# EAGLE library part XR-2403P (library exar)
Enhanced MNP-5 modem MICROCONTROLLER
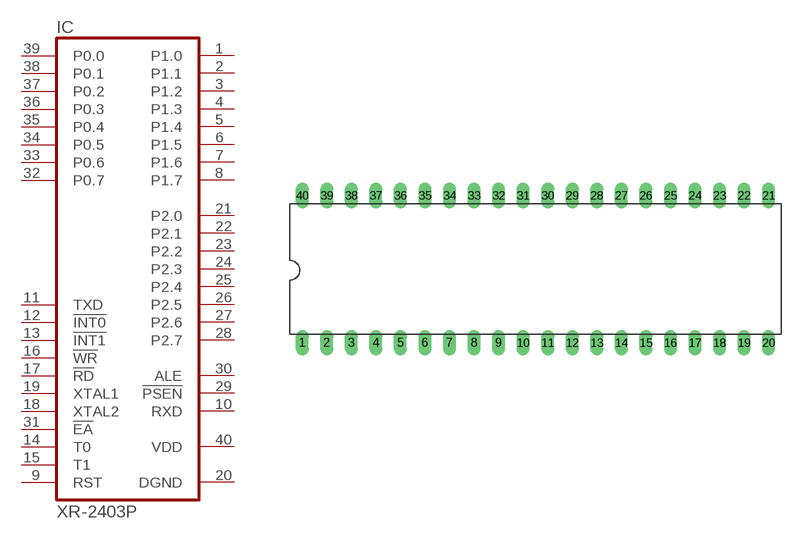
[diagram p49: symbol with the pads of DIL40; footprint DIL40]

Designator prefix IC

## XR-2403P (OC_FARNELL: unknown; OC_NEWARK: unknown)  [DIL40]
1  P1.0
2  P1.1
3  P1.2
4  P1.3
5  P1.4
6  P1.5
7  P1.6
8  P1.7
9  RST  in
10  RXD  out
11  TXD  in
12  !INT0  in
13  !INT1  in
14  T0  in
15  T1  in
16  !WR  in
17  !RD  in
18  XTAL2  in
19  XTAL1  in
20  DGND  pwr
21  P2.0
22  P2.1
23  P2.2
24  P2.3
25  P2.4
26  P2.5
27  P2.6
28  P2.7
29  !PSEN  out
30  ALE  out
31  !EA  in
32  P0.7
33  P0.6
34  P0.5
35  P0.4
36  P0.3
37  P0.2
38  P0.1
39  P0.0
40  VDD  pwr

## Footprint DIL40 (pad centres in mm)
Dual In Line Package
drill 0.813 long: 1 -24.13,-7.62; 2 -21.59,-7.62; 3 -19.05,-7.62; 4 -16.51,-7.62; 5 -13.97,-7.62; 6 -11.43,-7.62; 7 -8.89,-7.62; 8 -6.35,-7.62; 9 -3.81,-7.62; 10 -1.27,-7.62; 11 1.27,-7.62; 12 3.81,-7.62; 13 6.35,-7.62; 14 8.89,-7.62; 15 11.43,-7.62; 16 13.97,-7.62; 17 16.51,-7.62; 18 19.05,-7.62; 19 21.59,-7.62; 20 24.13,-7.62; 21 24.13,7.62; 22 21.59,7.62; 23 19.05,7.62; 24 16.51,7.62; 25 13.97,7.62; 26 11.43,7.62; 27 8.89,7.62; 28 6.35,7.62; 29 3.81,7.62; 30 1.27,7.62; 31 -1.27,7.62; 32 -3.81,7.62; 33 -6.35,7.62; 34 -8.89,7.62; 35 -11.43,7.62; 36 -13.97,7.62; 37 -16.51,7.62; 38 -19.05,7.62; 39 -21.59,7.62; 40 -24.13,7.62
